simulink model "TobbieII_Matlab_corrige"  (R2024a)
settings: Solver=VariableStepAuto  StartTime=0.0  StopTime=10  RelTol=1e-3
model workspace: external: MATLAB File (data not in the file)
undefined symbols (not defined in the file or in its folder): deg, kg, m, mm, N, s, smiData, X, Y, Z
libraries: sm_lib x63, fl_lib x16, nesl_utility x9, ee_lib x2, simulink x1
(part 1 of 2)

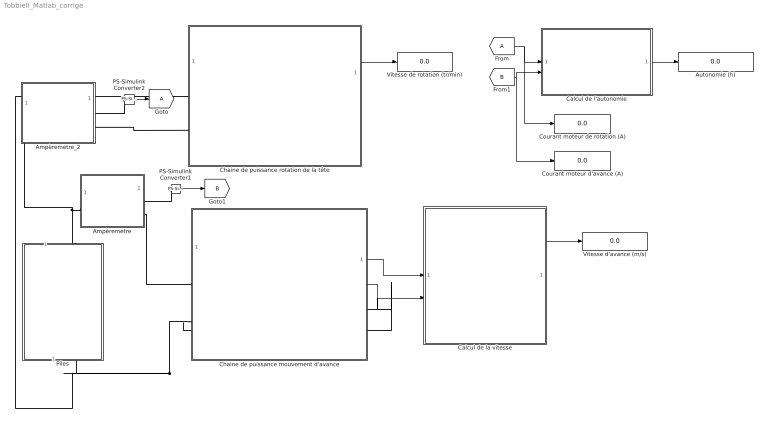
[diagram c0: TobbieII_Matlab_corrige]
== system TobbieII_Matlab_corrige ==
  Ampèremetre : Subsystem
  Ampèremetre_2 : Subsystem
  Autonomie (h) : Display
  Calcul de l'autonomie : Subsystem
  Calcul de la vitesse : Subsystem
  Chaine de puissance mouvement d'avance : Subsystem  mask{reducteur=(36*40*36*25)/(8*14*10*10)}
      mask prompts: reducteur "Rapport de réduction (1/r)"
  Chaine de puissance rotation de la tête : Subsystem  mask{reducteur=(34*32*36*32*60)/(8*14*10*14*10)}
      mask prompts: reducteur "rapport de reduction (1/r)"
  Courant moteur d'avance (A) : Display
  Courant moteur de rotation (A) : Display
  From : From
  Goto : Goto
  PS-Simulink Converter1 : nesl_utility/PS-Simulink Converter  PhysicalDomain=network_engine_domain  SubClassName=ps_output  LeftPortType=input  RightPortType=output  PseudoPeriodic=off  Frequencies=[]  VectorFormat=inherit  Unit=A  AffineConversion=off
  PS-Simulink Converter2 : nesl_utility/PS-Simulink Converter  PhysicalDomain=network_engine_domain  SubClassName=ps_output  LeftPortType=input  RightPortType=output  PseudoPeriodic=off  Frequencies=[]  VectorFormat=inherit  Unit=A  AffineConversion=off
  Piles : Subsystem  mask{tension=6}
      mask prompts: tension "Tension (V)"
  Vitesse d'avance (m/s) : Display
  Vitesse de rotation (tr/min) : Display
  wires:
  Calcul de la vitesse/1(v) -> Vitesse d'avance (m/s)/1
  PS-Simulink Converter1/1 -> [B]
  PS-Simulink Converter2/1 -> Goto/1
  Chaine de puissance mouvement d'avance/1(G2x) -> Calcul de la vitesse/1(In1)
  Chaine de puissance mouvement d'avance/2(G1x) -> Calcul de la vitesse/2(In2)
  From/1 -> Courant moteur de rotation (A)/1, Calcul de l'autonomie/1(In1)
  [B] -> Courant moteur d'avance (A)/1, Calcul de l'autonomie/2(In2)
  Calcul de l'autonomie/1(Out1) -> Autonomie (h)/1
  Chaine de puissance rotation de la tête/1(Out1) -> Vitesse de rotation (tr/min)/1
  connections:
  Ampèremetre/LConn1 -- Ampèremetre_2/LConn1 -- Piles/LConn1
  PS-Simulink Converter1/LConn1 -- Ampèremetre/RConn1
  Ampèremetre/RConn2 -- Chaine de puissance mouvement d'avance/LConn1
  PS-Simulink Converter2/LConn1 -- Ampèremetre_2/RConn1
  Ampèremetre_2/RConn2 -- Chaine de puissance rotation de la tête/LConn2
  Chaine de puissance mouvement d'avance/LConn2 -- Piles/RConn1 -- Chaine de puissance rotation de la tête/LConn1 -- Chaine de puissance mouvement d'avance/RConn1

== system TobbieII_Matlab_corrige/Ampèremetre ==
  Current Sensor : fl_lib/Electrical/Electrical Sensors/Current Sensor
  Conn1 : PMIOPort  Side=Right
  Conn2 : PMIOPort  Port=2  Side=Left
  Conn3 : PMIOPort  Port=3  Side=Right
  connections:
  Current Sensor/LConn1 -- Conn2/RConn1
  Conn1/RConn1 -- Current Sensor/RConn1
  Current Sensor/RConn2 -- Conn3/RConn1

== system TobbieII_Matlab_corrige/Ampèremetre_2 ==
  Current Sensor1 : fl_lib/Electrical/Electrical Sensors/Current Sensor
  Conn1 : PMIOPort  Side=Left
  Conn2 : PMIOPort  Port=2  Side=Right
  Conn3 : PMIOPort  Port=3  Side=Right
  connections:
  Conn2/RConn1 -- Current Sensor1/RConn1
  Current Sensor1/LConn1 -- Conn1/RConn1
  Current Sensor1/RConn2 -- Conn3/RConn1

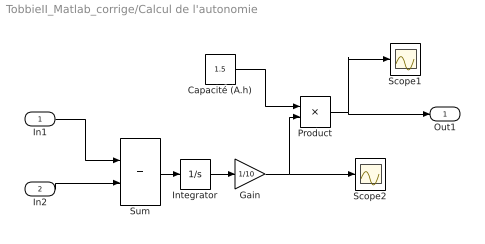
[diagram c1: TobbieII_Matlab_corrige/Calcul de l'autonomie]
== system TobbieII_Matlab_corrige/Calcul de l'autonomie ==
  In1 : Inport
  In2 : Inport  Port=2
  Capacité (A.h) : Constant  Value=1.5
  Gain : Gain  Gain=1/10
  Integrator : Integrator
  Product : Product  Inputs=*/
  Scope1 : Scope
  Scope2 : Scope
  Sum : Sum
  Out1 : Outport
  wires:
  Integrator/1 -> Gain/1
  Gain/1 -> Scope2/1, Product/2
  Capacité (A.h)/1 -> Product/1
  Sum/1 -> Integrator/1
  Product/1 -> Out1/1, Scope1/1
  In1/1 -> Sum/1
  In2/1 -> Sum/2

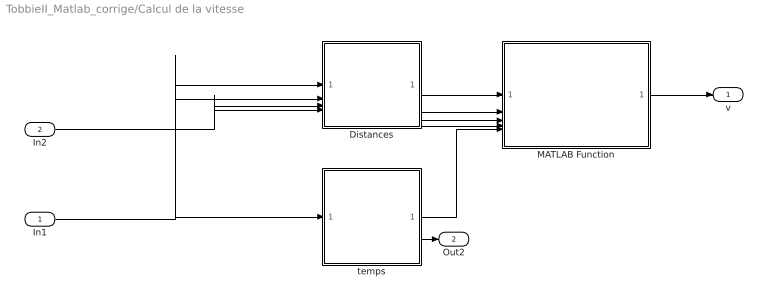
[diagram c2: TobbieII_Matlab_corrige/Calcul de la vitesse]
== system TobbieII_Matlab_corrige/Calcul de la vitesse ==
  In1 : Inport
  In2 : Inport  Port=2
  Distances : Subsystem
  MATLAB Function : MATLAB Function  TreatAsAtomicUnit=on
  temps : Subsystem
  v : Outport
  Out2 : Outport  Port=2
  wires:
  Distances/3(Out3) -> MATLAB Function/3(G2xMax)
  Distances/1(Out1) -> MATLAB Function/1(G1xMax)
  Distances/4(Out4) -> MATLAB Function/4(G2xMin)
  In2/1 -> Distances/4(In4), Distances/3(In3)
  In1/1 -> Distances/1(In1), Distances/2(In2), temps/1(U)
  temps/2(Out2) -> Out2/1
  Distances/2(Out2) -> MATLAB Function/2(G1xMin)
  temps/1(Out1) -> MATLAB Function/5(t)
  MATLAB Function/1(v) -> v/1

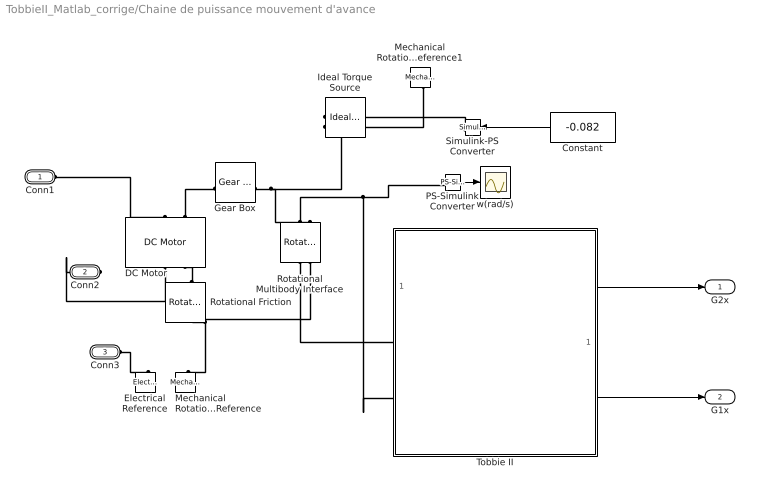
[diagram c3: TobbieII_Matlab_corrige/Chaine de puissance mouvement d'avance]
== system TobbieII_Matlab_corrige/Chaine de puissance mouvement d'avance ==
  Constant : Constant  Value=-0.082
  DC Motor : ee_lib/Electromechanical/Brushed Motors/DC Motor  field_option=ee.enum.field_option.pm  Rf=100 Ohm  Lf=1 H  Laf=0.15 H  If0=0 A  parameterization=ee.enum.dcparam_option.circuit_param  Ra=6.18 Ohm  La=2 mH  emf_or_torque=ee.enum.emf_or_torque.kv  Kv=0.0042 V*s/rad  Ki=6.876e-4 N*m/A  T_stall=0.24e-3 N*m  w_max=19100 rpm  w_rated=15000 rpm  P_rated=0.08 W  V_rated=1.5 V  lam_param=ee.enum.lam_param.damping  i_noload=0 A  V_i_noload=1.5 V  J=0.01 cm^2*g  lam=0 N*m*s/rad  speed0=0 rpm  enable_fault_armature=simscape.enum.onoff.off  rev_faulted=1 / 3  G_faulted_armature=1e-5 S  fault_trigger_armature=ee.enum.faults.faultTrigger.temporal  t_fault_armature=1 s  max_permissible_current_armature=inf A  t_fail_on_current_armature=1 s  enable_fault_field=simscape.enum.onoff.off  G_faulted_field=1e-5 S  fault_trigger_field=ee.enum.faults.faultTrigger.temporal  t_fault_field=1 s  max_permissible_current_field=inf A  t_fail_on_current_field=1 s  fault_action=simscape.enum.assert.action.none  alpha=3.93e-3 1/K  Tmeas=25 degC  thermal_mass=100 J/K  initial_temperature=25 degC
  Electrical Reference : fl_lib/Electrical/Electrical Elements/Electrical Reference
  Gear Box : fl_lib/Mechanical/Mechanisms/Gear Box  ratio=reducteur  t_in_specify=off  t_in_priority=None  t_in=0 N*m  t_in_nominal_specify=off  t_in_nominal_value=1  t_in_nominal_unit=N*m  t_out_specify=off  t_out_priority=None  t_out=0 N*m  t_out_nominal_specify=off  t_out_nominal_value=1  t_out_nominal_unit=N*m
  Ideal Torque Source : fl_lib/Mechanical/Mechanical Sources/Ideal Torque Source
  Mechanical Rotational Reference : fl_lib/Mechanical/Rotational Elements/Mechanical Rotational Reference
  Mechanical Rotational Reference1 : fl_lib/Mechanical/Rotational Elements/Mechanical Rotational Reference
  PS-Simulink Converter : nesl_utility/PS-Simulink Converter  PhysicalDomain=network_engine_domain  SubClassName=ps_output  LeftPortType=input  RightPortType=output  PseudoPeriodic=off  Frequencies=[]  VectorFormat=inherit  Unit=inherit  AffineConversion=off
  Rotational Friction : fl_lib/Mechanical/Rotational Elements/Rotational Friction  brkwy_trq=0.0029*0.007*1.8 N*m  brkwy_vel=0.01 rad/s  Col_trq=0.0029*0.005 N*m  visc_coef=0.0029*(0.14-0.007)/1365 N*m*s/rad  w_specify=off  w_priority=None  w=0 rad/s  w_nominal_specify=off  w_nominal_value=1  w_nominal_unit=rad/s  t_specify=off  t_priority=None  t=0 N*m  t_nominal_specify=off  t_nominal_value=1  t_nominal_unit=N*m
  Rotational Multibody Interface : fl_lib/Mechanical/Multibody Interfaces/Rotational Multibody Interface
  Simulink-PS Converter : nesl_utility/Simulink-PS Converter  PhysicalDomain=network_engine_domain  SubClassName=ps_input  LeftPortType=input  RightPortType=output  PseudoPeriodic=off  Frequencies=[]  NoiseDistribution=none  NoiseParameters=[]  Unit=N*m  AffineConversion=off  FilteringAndDerivatives=provide  SimscapeFilterOrder=1  InputFilterTimeConstant=0.001  UdotUserProvided=0
  Tobbie II : Subsystem
  w(rad/s) : Scope
  Conn1 : PMIOPort  Side=Left
  Conn2 : PMIOPort  Port=2  Side=Right
  Conn3 : PMIOPort  Port=3  Side=Left
  G2x : Outport
  G1x : Outport  Port=2
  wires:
  Constant/1 -> Simulink-PS Converter/1
  PS-Simulink Converter/1 -> w(rad/s)/1
  Tobbie II/2(G1x) -> G1x/1
  Tobbie II/1(G2x) -> G2x/1
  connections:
  Rotational Friction/RConn1 -- DC Motor/RConn2
  Gear Box/RConn1 -- Ideal Torque Source/LConn1 -- Rotational Multibody Interface/RConn2
  Rotational Multibody Interface/RConn1 -- PS-Simulink Converter/LConn1 -- Tobbie II/LConn2
  DC Motor/LConn2 -- Gear Box/LConn1
  Rotational Multibody Interface/LConn2 -- Rotational Friction/LConn1 -- Mechanical Rotational Reference/LConn1
  Rotational Multibody Interface/LConn1 -- Tobbie II/LConn1
  Mechanical Rotational Reference1/LConn1 -- Ideal Torque Source/RConn2
  Simulink-PS Converter/RConn1 -- Ideal Torque Source/RConn1
  Conn1/RConn1 -- DC Motor/LConn1
  DC Motor/RConn1 -- Conn2/RConn1
  Conn3/RConn1 -- Electrical Reference/LConn1

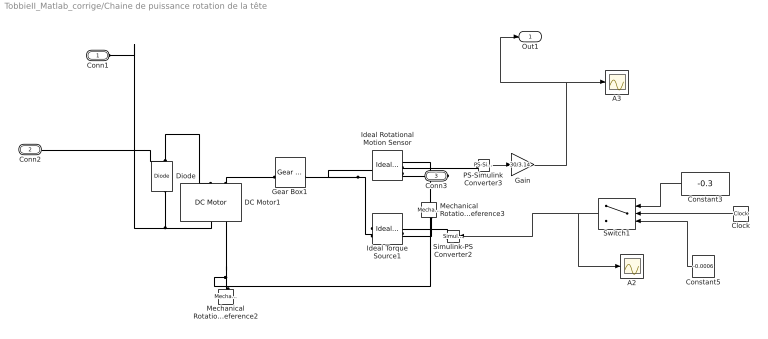
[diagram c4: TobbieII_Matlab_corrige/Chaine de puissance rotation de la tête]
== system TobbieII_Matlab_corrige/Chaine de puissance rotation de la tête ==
  A2 : Scope
  A3 : Scope
  Clock : Clock
  Constant3 : Constant  Value=-0.3
  Constant5 : Constant  Value=-0.0006
  DC Motor1 : ee_lib/Electromechanical/Brushed Motors/DC Motor  field_option=ee.enum.field_option.pm  Rf=100 Ohm  Lf=1 H  Laf=0.15 H  If0=0 A  parameterization=ee.enum.dcparam_option.circuit_param  Ra=6.18 Ohm  La=2 mH  emf_or_torque=ee.enum.emf_or_torque.kv  Kv=0.0045 V*s/rad  Ki=6.876e-4 N*m/A  T_stall=0.24e-3 N*m  w_max=19100 rpm  w_rated=15000 rpm  P_rated=0.08 W  V_rated=1.5 V  lam_param=ee.enum.lam_param.damping  i_noload=0 A  V_i_noload=1.5 V  J=0.00001 cm^2*g  lam=0 N*m*s/rad  speed0=0 rpm  enable_fault_armature=simscape.enum.onoff.off  rev_faulted=1 / 3  G_faulted_armature=1e-5 S  fault_trigger_armature=ee.enum.faults.faultTrigger.temporal  t_fault_armature=1 s  max_permissible_current_armature=inf A  t_fail_on_current_armature=1 s  enable_fault_field=simscape.enum.onoff.off  G_faulted_field=1e-5 S  fault_trigger_field=ee.enum.faults.faultTrigger.temporal  t_fault_field=1 s  max_permissible_current_field=inf A  t_fail_on_current_field=1 s  fault_action=simscape.enum.assert.action.none  alpha=3.93e-3 1/K  Tmeas=25 degC  thermal_mass=100 J/K  initial_temperature=25 degC
  Diode : fl_lib/Electrical/Electrical Elements/Diode  Vf=0.6 V  Ron=0.3 Ohm  Goff=1e-8 1/Ohm  i_specify=off  i_priority=None  i=0 A  i_nominal_specify=off  i_nominal_value=1  i_nominal_unit=A  v_specify=off  v_priority=None  v=0 V  v_nominal_specify=off  v_nominal_value=1  v_nominal_unit=V
  Gain : Gain  Gain=30/3.14
  Gear Box1 : fl_lib/Mechanical/Mechanisms/Gear Box  ratio=reducteur  t_in_specify=off  t_in_priority=None  t_in=0 N*m  t_in_nominal_specify=off  t_in_nominal_value=1  t_in_nominal_unit=N*m  t_out_specify=off  t_out_priority=None  t_out=0 N*m  t_out_nominal_specify=off  t_out_nominal_value=1  t_out_nominal_unit=N*m
  Ideal Rotational Motion Sensor : fl_lib/Mechanical/Mechanical Sensors/Ideal Rotational Motion Sensor  reference=foundation.enum.MeasurementReference.difference  acceleration_port=false  velocity_port=true  position_port=true  wrap_angle=false  offset=0 rad
  Ideal Torque Source1 : fl_lib/Mechanical/Mechanical Sources/Ideal Torque Source
  Mechanical Rotational Reference2 : fl_lib/Mechanical/Rotational Elements/Mechanical Rotational Reference
  Mechanical Rotational Reference3 : fl_lib/Mechanical/Rotational Elements/Mechanical Rotational Reference
  PS-Simulink Converter3 : nesl_utility/PS-Simulink Converter  PhysicalDomain=network_engine_domain  SubClassName=ps_output  LeftPortType=input  RightPortType=output  PseudoPeriodic=off  Frequencies=[]  VectorFormat=inherit  Unit=rad/s  AffineConversion=off
  Simulink-PS Converter2 : nesl_utility/Simulink-PS Converter  PhysicalDomain=network_engine_domain  SubClassName=ps_input  LeftPortType=input  RightPortType=output  PseudoPeriodic=off  Frequencies=[]  NoiseDistribution=none  NoiseParameters=[]  Unit=N*m  AffineConversion=off  FilteringAndDerivatives=provide  SimscapeFilterOrder=1  InputFilterTimeConstant=0.001  UdotUserProvided=0
  Switch1 : Switch  Criteria=u2 > Threshold  Threshold=7
  Conn1 : PMIOPort  Side=Left
  Conn2 : PMIOPort  Port=2  Side=Left
  Conn3 : PMIOPort  Port=3  Side=Right
  Out1 : Outport
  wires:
  Switch1/1 -> A2/1, Simulink-PS Converter2/1
  Clock/1 -> Switch1/2
  Constant5/1 -> Switch1/3
  Constant3/1 -> Switch1/1
  PS-Simulink Converter3/1 -> Gain/1
  Gain/1 -> Out1/1, A3/1
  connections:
  Diode/RConn1 -- Conn2/RConn1 -- DC Motor1/LConn1
  Ideal Torque Source1/LConn1 -- Ideal Rotational Motion Sensor/LConn1 -- Gear Box1/RConn1
  Mechanical Rotational Reference3/LConn1 -- Ideal Torque Source1/RConn2
  Mechanical Rotational Reference2/LConn1 -- DC Motor1/RConn2 -- Ideal Rotational Motion Sensor/RConn1
  Diode/LConn1 -- Conn1/RConn1 -- DC Motor1/RConn1
  PS-Simulink Converter3/LConn1 -- Ideal Rotational Motion Sensor/RConn2
  Ideal Rotational Motion Sensor/RConn3 -- Conn3/RConn1
  DC Motor1/LConn2 -- Gear Box1/LConn1
  Simulink-PS Converter2/RConn1 -- Ideal Torque Source1/RConn1

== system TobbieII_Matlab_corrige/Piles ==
  DC Voltage Source1 : fl_lib/Electrical/Electrical Sources/DC Voltage Source  v0=tension V
  Conn1 : PMIOPort  Side=Left
  Conn2 : PMIOPort  Port=2  Side=Right
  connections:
  DC Voltage Source1/RConn1 -- Conn2/RConn1
  Conn1/RConn1 -- DC Voltage Source1/LConn1

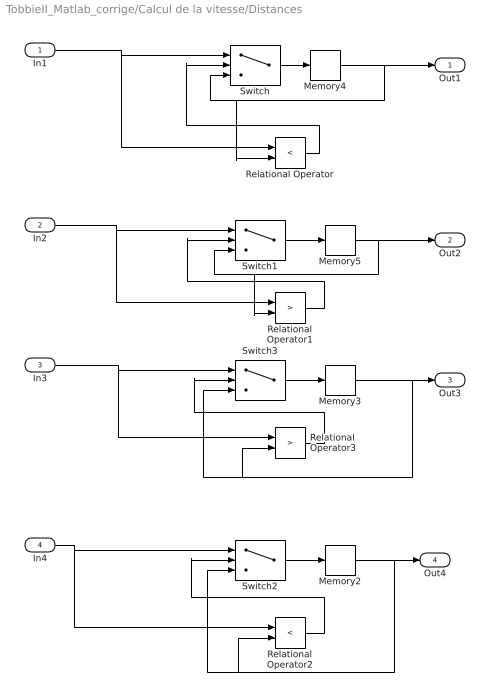
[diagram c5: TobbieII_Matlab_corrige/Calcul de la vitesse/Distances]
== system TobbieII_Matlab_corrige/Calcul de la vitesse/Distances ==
  In1 : Inport
  In2 : Inport  Port=2
  In3 : Inport  Port=3
  In4 : Inport  Port=4
  Memory2 : Memory  InitialCondition=0.09
  Memory3 : Memory  InitialCondition=0.09
  Memory4 : Memory  InitialCondition=-0.04
  Memory5 : Memory  InitialCondition=-0.04
  Relational Operator : RelationalOperator  Operator=<  OutDataTypeStr=boolean  RndMeth=Simplest
  Relational Operator1 : RelationalOperator  Operator=>  OutDataTypeStr=boolean  RndMeth=Simplest
  Relational Operator2 : RelationalOperator  Operator=<  OutDataTypeStr=boolean  RndMeth=Simplest
  Relational Operator3 : RelationalOperator  Operator=>  OutDataTypeStr=boolean  RndMeth=Simplest
  Switch{,1..3} (4 alike) : Switch  Criteria=u2 > Threshold
  Out1 : Outport
  Out2 : Outport  Port=2
  Out3 : Outport  Port=3
  Out4 : Outport  Port=4
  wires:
  Memory5/1 -> Relational Operator1/2, Switch1/3, Out2/1
  Relational Operator3/1 -> Switch3/2
  Memory3/1 -> Switch3/3, Relational Operator3/2, Out3/1
  Switch/1 -> Memory4/1
  In4/1 -> Relational Operator2/1, Switch2/1
  In1/1 -> Relational Operator/1, Switch/1
  Switch3/1 -> Memory3/1
  Memory4/1 -> Relational Operator/2, Switch/3, Out1/1
  In2/1 -> Relational Operator1/1, Switch1/1
  In3/1 -> Relational Operator3/1, Switch3/1
  Switch1/1 -> Memory5/1
  Memory2/1 -> Switch2/3, Relational Operator2/2, Out4/1
  Relational Operator/1 -> Switch/2
  Relational Operator2/1 -> Switch2/2
  Relational Operator1/1 -> Switch1/2
  Switch2/1 -> Memory2/1

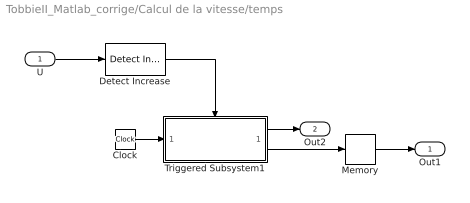
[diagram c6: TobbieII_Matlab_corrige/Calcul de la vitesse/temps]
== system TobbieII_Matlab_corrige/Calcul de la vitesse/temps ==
  U : Inport
  Clock : Clock
  Detect Increase : simulink/Logic and Bit Operations/Detect Increase  vinit=0.0  OutDataTypeStr=boolean
  Memory : Memory
  Triggered Subsystem1 : Subsystem  TreatAsAtomicUnit=on
  Out1 : Outport
  Out2 : Outport  Port=2
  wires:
  Triggered Subsystem1/2(Out2) -> Memory/1
  Memory/1 -> Out1/1
  Detect Increase/1 -> Triggered Subsystem1/Trigger
  Clock/1 -> Triggered Subsystem1/1(In1)
  Triggered Subsystem1/1(Out1) -> Out2/1
  U/1 -> Detect Increase/1

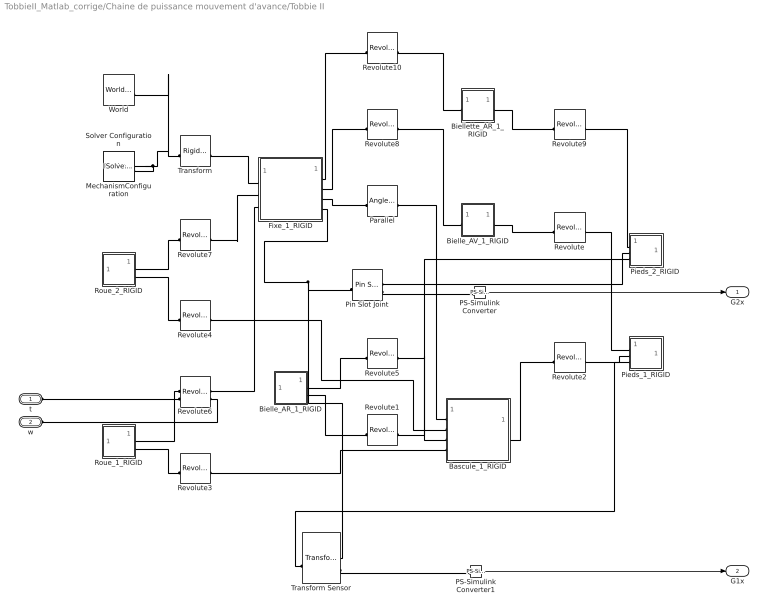
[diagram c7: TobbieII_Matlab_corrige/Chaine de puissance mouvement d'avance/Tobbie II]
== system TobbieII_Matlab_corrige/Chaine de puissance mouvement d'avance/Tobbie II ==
  Bascule_1_RIGID : Subsystem
  Bielle_AR_1_RIGID : Subsystem
  Bielle_AV_1_RIGID : Subsystem
  Biellette_AR_1_RIGID : Subsystem
  Fixe_1_RIGID : Subsystem
  MechanismConfiguration : sm_lib/Utilities/Mechanism Configuration  UniformGravity=Constant  GravityVector=[0 -9.80665 0]  GravityVectorUnits=m/s^2  LinearizationDelta=0.001  JointModeTransitionNonlinearIterations=2
  PS-Simulink Converter : nesl_utility/PS-Simulink Converter  PhysicalDomain=network_engine_domain  SubClassName=ps_output  LeftPortType=input  RightPortType=output  PseudoPeriodic=off  Frequencies=[]  VectorFormat=inherit  Unit=m  AffineConversion=off
  PS-Simulink Converter1 : nesl_utility/PS-Simulink Converter  PhysicalDomain=network_engine_domain  SubClassName=ps_output  LeftPortType=input  RightPortType=output  PseudoPeriodic=off  Frequencies=[]  VectorFormat=inherit  Unit=m  AffineConversion=off
  Parallel : sm_lib/Constraints/Angle Constraint  ConstraintType=Parallel  Angle=45  AngleUnits=deg  WrenchDir=FollowerOnBase  WrenchFrame=BaseFrame  SenseTorque=off  SenseSignedTorqueMagnitude=off
  Pieds_1_RIGID : Subsystem
  Pieds_2_RIGID : Subsystem
  Pin Slot Joint : sm_lib/Joints/Pin Slot Joint  JointMode=Normal  CompositeWrenchDir=FollowerOnBase  CompositeWrenchFrame=BaseFrame  SenseConstraintForce=off  SenseConstraintTorque=off  SenseTotalForce=off  SenseTotalTorque=off  PxPositionTargetSpecify=off  PxPositionTargetPriority=High  PxPositionTargetValue=0  PxPositionTargetValueUnits=m  PxVelocityTargetSpecify=off  PxVelocityTargetPriority=High  PxVelocityTargetValue=0  PxVelocityTargetValueUnits=m/s  PxEquilibriumPosition=0  PxEquilibriumPositionUnits=m  PxSpringStiffness=0  PxSpringStiffnessUnits=N/m  PxDampingCoefficient=0  PxDampingCoefficientUnits=N/(m/s)  PxLowerLimitSpecify=off  PxLowerLimitBound=-1  PxLowerLimitBoundUnits=m  PxLowerLimitStiffness=1e6  PxLowerLimitStiffnessUnits=N/m  PxLowerLimitDamping=1e3  PxLowerLimitDampingUnits=N/(m/s)  PxLowerLimitTransitionRegionWidth=1e-4  PxLowerLimitTransitionRegionWidthUnits=m  PxUpperLimitSpecify=off  PxUpperLimitBound=1  PxUpperLimitBoundUnits=m  PxUpperLimitStiffness=1e6  PxUpperLimitStiffnessUnits=N/m  PxUpperLimitDamping=1e3  PxUpperLimitDampingUnits=N/(m/s)  PxUpperLimitTransitionRegionWidth=1e-4  PxUpperLimitTransitionRegionWidthUnits=m  PxTorqueActuationMode=NoTorque  PxMotionActuationMode=ComputedMotion  PxSensePosition=on  PxSenseVelocity=off  PxSenseAcceleration=off  PxSenseTorqueForce=off  PxSenseLowerLimitTorqueForce=off  PxSenseUpperLimitTorqueForce=off  RzPositionTargetSpecify=off  RzPositionTargetPriority=High  RzPositionTargetValue=0  RzPositionTargetValueUnits=deg  RzVelocityTargetSpecify=off  RzVelocityTargetPriority=High  RzVelocityTargetValue=0  RzVelocityTargetValueUnits=deg/s  RzEquilibriumPosition=0  RzEquilibriumPositionUnits=deg  RzSpringStiffness=0  RzSpringStiffnessUnits=N*m/deg  RzDampingCoefficient=0  RzDampingCoefficientUnits=N*m/(deg/s)  RzLowerLimitSpecify=off  RzLowerLimitBound=-90  RzLowerLimitBoundUnits=deg  RzLowerLimitStiffness=1e4  RzLowerLimitStiffnessUnits=N*m/deg  RzLowerLimitDamping=10  RzLowerLimitDampingUnits=N*m/(deg/s)  RzLowerLimitTransitionRegionWidth=0.1  RzLowerLimitTransitionRegionWidthUnits=deg  RzUpperLimitSpecify=off  RzUpperLimitBound=90  RzUpperLimitBoundUnits=deg  RzUpperLimitStiffness=1e4  RzUpperLimitStiffnessUnits=N*m/deg  RzUpperLimitDamping=10  RzUpperLimitDampingUnits=N*m/(deg/s)  RzUpperLimitTransitionRegionWidth=0.1  RzUpperLimitTransitionRegionWidthUnits=deg  RzTorqueActuationMode=NoTorque  RzMotionActuationMode=ComputedMotion  RzSensePosition=off  RzSenseVelocity=off  RzSenseAcceleration=off  RzSenseTorqueForce=off  RzSenseLowerLimitTorqueForce=off  RzSenseUpperLimitTorqueForce=off
  Revolute : sm_lib/Joints/Revolute Joint  JointMode=Normal  CompositeWrenchDir=FollowerOnBase  CompositeWrenchFrame=BaseFrame  SenseConstraintForce=off  SenseConstraintTorque=off  SenseTotalForce=off  SenseTotalTorque=off  PositionTargetSpecify=on  PositionTargetPriority=Low  PositionTargetValue=smiData.RevoluteJoint(1).Rz.Pos  PositionTargetValueUnits=deg  VelocityTargetSpecify=off  VelocityTargetPriority=High  VelocityTargetValue=0  VelocityTargetValueUnits=deg/s  EquilibriumPosition=0  EquilibriumPositionUnits=deg  SpringStiffness=0  SpringStiffnessUnits=N*m/deg  DampingCoefficient=0  DampingCoefficientUnits=N*m/(deg/s)  LowerLimitSpecify=off  LowerLimitBound=-90  LowerLimitBoundUnits=deg  LowerLimitStiffness=1e4  LowerLimitStiffnessUnits=N*m/deg  LowerLimitDamping=10  LowerLimitDampingUnits=N*m/(deg/s)  LowerLimitTransitionRegionWidth=0.1  LowerLimitTransitionRegionWidthUnits=deg  UpperLimitSpecify=off  UpperLimitBound=90  UpperLimitBoundUnits=deg  UpperLimitStiffness=1e4  UpperLimitStiffnessUnits=N*m/deg  UpperLimitDamping=10  UpperLimitDampingUnits=N*m/(deg/s)  UpperLimitTransitionRegionWidth=0.1  UpperLimitTransitionRegionWidthUnits=deg  TorqueActuationMode=NoTorque  MotionActuationMode=ComputedMotion  SensePosition=off  SenseVelocity=off  SenseAcceleration=off  SenseTorqueForce=off  SenseLowerLimitTorqueForce=off  SenseUpperLimitTorqueForce=off
  Revolute1 : sm_lib/Joints/Revolute Joint  JointMode=Normal  CompositeWrenchDir=FollowerOnBase  CompositeWrenchFrame=BaseFrame  SenseConstraintForce=off  SenseConstraintTorque=off  SenseTotalForce=off  SenseTotalTorque=off  PositionTargetSpecify=on  PositionTargetPriority=Low  PositionTargetValue=smiData.RevoluteJoint(2).Rz.Pos  PositionTargetValueUnits=deg  VelocityTargetSpecify=off  VelocityTargetPriority=High  VelocityTargetValue=0  VelocityTargetValueUnits=deg/s  EquilibriumPosition=0  EquilibriumPositionUnits=deg  SpringStiffness=0  SpringStiffnessUnits=N*m/deg  DampingCoefficient=0  DampingCoefficientUnits=N*m/(deg/s)  LowerLimitSpecify=off  LowerLimitBound=-90  LowerLimitBoundUnits=deg  LowerLimitStiffness=1e4  LowerLimitStiffnessUnits=N*m/deg  LowerLimitDamping=10  LowerLimitDampingUnits=N*m/(deg/s)  LowerLimitTransitionRegionWidth=0.1  LowerLimitTransitionRegionWidthUnits=deg  UpperLimitSpecify=off  UpperLimitBound=90  UpperLimitBoundUnits=deg  UpperLimitStiffness=1e4  UpperLimitStiffnessUnits=N*m/deg  UpperLimitDamping=10  UpperLimitDampingUnits=N*m/(deg/s)  UpperLimitTransitionRegionWidth=0.1  UpperLimitTransitionRegionWidthUnits=deg  TorqueActuationMode=NoTorque  MotionActuationMode=ComputedMotion  SensePosition=off  SenseVelocity=off  SenseAcceleration=off  SenseTorqueForce=off  SenseLowerLimitTorqueForce=off  SenseUpperLimitTorqueForce=off
  Revolute10 : sm_lib/Joints/Revolute Joint  JointMode=Normal  CompositeWrenchDir=FollowerOnBase  CompositeWrenchFrame=BaseFrame  SenseConstraintForce=off  SenseConstraintTorque=off  SenseTotalForce=off  SenseTotalTorque=off  PositionTargetSpecify=on  PositionTargetPriority=Low  PositionTargetValue=smiData.RevoluteJoint(11).Rz.Pos  PositionTargetValueUnits=deg  VelocityTargetSpecify=off  VelocityTargetPriority=High  VelocityTargetValue=0  VelocityTargetValueUnits=deg/s  EquilibriumPosition=0  EquilibriumPositionUnits=deg  SpringStiffness=0  SpringStiffnessUnits=N*m/deg  DampingCoefficient=0  DampingCoefficientUnits=N*m/(deg/s)  LowerLimitSpecify=off  LowerLimitBound=-90  LowerLimitBoundUnits=deg  LowerLimitStiffness=1e4  LowerLimitStiffnessUnits=N*m/deg  LowerLimitDamping=10  LowerLimitDampingUnits=N*m/(deg/s)  LowerLimitTransitionRegionWidth=0.1  LowerLimitTransitionRegionWidthUnits=deg  UpperLimitSpecify=off  UpperLimitBound=90  UpperLimitBoundUnits=deg  UpperLimitStiffness=1e4  UpperLimitStiffnessUnits=N*m/deg  UpperLimitDamping=10  UpperLimitDampingUnits=N*m/(deg/s)  UpperLimitTransitionRegionWidth=0.1  UpperLimitTransitionRegionWidthUnits=deg  TorqueActuationMode=NoTorque  MotionActuationMode=ComputedMotion  SensePosition=off  SenseVelocity=off  SenseAcceleration=off  SenseTorqueForce=off  SenseLowerLimitTorqueForce=off  SenseUpperLimitTorqueForce=off
  Revolute{2,4..5,9} (4 alike) : sm_lib/Joints/Revolute Joint  JointMode=Normal  CompositeWrenchDir=FollowerOnBase  CompositeWrenchFrame=BaseFrame  SenseConstraintForce=off  SenseConstraintTorque=off  SenseTotalForce=off  SenseTotalTorque=off  PositionTargetSpecify=off  PositionTargetPriority=High  PositionTargetValue=0  PositionTargetValueUnits=deg  VelocityTargetSpecify=off  VelocityTargetPriority=High  VelocityTargetValue=0  VelocityTargetValueUnits=deg/s  EquilibriumPosition=0  EquilibriumPositionUnits=deg  SpringStiffness=0  SpringStiffnessUnits=N*m/deg  DampingCoefficient=0  DampingCoefficientUnits=N*m/(deg/s)  LowerLimitSpecify=off  LowerLimitBound=-90  LowerLimitBoundUnits=deg  LowerLimitStiffness=1e4  LowerLimitStiffnessUnits=N*m/deg  LowerLimitDamping=10  LowerLimitDampingUnits=N*m/(deg/s)  LowerLimitTransitionRegionWidth=0.1  LowerLimitTransitionRegionWidthUnits=deg  UpperLimitSpecify=off  UpperLimitBound=90  UpperLimitBoundUnits=deg  UpperLimitStiffness=1e4  UpperLimitStiffnessUnits=N*m/deg  UpperLimitDamping=10  UpperLimitDampingUnits=N*m/(deg/s)  UpperLimitTransitionRegionWidth=0.1  UpperLimitTransitionRegionWidthUnits=deg  TorqueActuationMode=NoTorque  MotionActuationMode=ComputedMotion  SensePosition=off  SenseVelocity=off  SenseAcceleration=off  SenseTorqueForce=off  SenseLowerLimitTorqueForce=off  SenseUpperLimitTorqueForce=off
  Revolute3 : sm_lib/Joints/Revolute Joint  JointMode=Normal  CompositeWrenchDir=FollowerOnBase  CompositeWrenchFrame=BaseFrame  SenseConstraintForce=off  SenseConstraintTorque=off  SenseTotalForce=off  SenseTotalTorque=off  PositionTargetSpecify=on  PositionTargetPriority=Low  PositionTargetValue=smiData.RevoluteJoint(4).Rz.Pos  PositionTargetValueUnits=deg  VelocityTargetSpecify=off  VelocityTargetPriority=High  VelocityTargetValue=0  VelocityTargetValueUnits=deg/s  EquilibriumPosition=0  EquilibriumPositionUnits=deg  SpringStiffness=0  SpringStiffnessUnits=N*m/deg  DampingCoefficient=0  DampingCoefficientUnits=N*m/(deg/s)  LowerLimitSpecify=off  LowerLimitBound=-90  LowerLimitBoundUnits=deg  LowerLimitStiffness=1e4  LowerLimitStiffnessUnits=N*m/deg  LowerLimitDamping=10  LowerLimitDampingUnits=N*m/(deg/s)  LowerLimitTransitionRegionWidth=0.1  LowerLimitTransitionRegionWidthUnits=deg  UpperLimitSpecify=off  UpperLimitBound=90  UpperLimitBoundUnits=deg  UpperLimitStiffness=1e4  UpperLimitStiffnessUnits=N*m/deg  UpperLimitDamping=10  UpperLimitDampingUnits=N*m/(deg/s)  UpperLimitTransitionRegionWidth=0.1  UpperLimitTransitionRegionWidthUnits=deg  TorqueActuationMode=NoTorque  MotionActuationMode=ComputedMotion  SensePosition=off  SenseVelocity=off  SenseAcceleration=off  SenseTorqueForce=off  SenseLowerLimitTorqueForce=off  SenseUpperLimitTorqueForce=off
  Revolute6 : sm_lib/Joints/Revolute Joint  JointMode=Normal  CompositeWrenchDir=FollowerOnBase  CompositeWrenchFrame=BaseFrame  SenseConstraintForce=off  SenseConstraintTorque=off  SenseTotalForce=off  SenseTotalTorque=off  PositionTargetSpecify=on  PositionTargetPriority=Low  PositionTargetValue=smiData.RevoluteJoint(7).Rz.Pos  PositionTargetValueUnits=deg  VelocityTargetSpecify=off  VelocityTargetPriority=High  VelocityTargetValue=0  VelocityTargetValueUnits=deg/s  EquilibriumPosition=0  EquilibriumPositionUnits=deg  SpringStiffness=0  SpringStiffnessUnits=N*m/deg  DampingCoefficient=0  DampingCoefficientUnits=N*m/(deg/s)  LowerLimitSpecify=off  LowerLimitBound=-90  LowerLimitBoundUnits=deg  LowerLimitStiffness=1e4  LowerLimitStiffnessUnits=N*m/deg  LowerLimitDamping=10  LowerLimitDampingUnits=N*m/(deg/s)  LowerLimitTransitionRegionWidth=0.1  LowerLimitTransitionRegionWidthUnits=deg  UpperLimitSpecify=off  UpperLimitBound=90  UpperLimitBoundUnits=deg  UpperLimitStiffness=1e4  UpperLimitStiffnessUnits=N*m/deg  UpperLimitDamping=10  UpperLimitDampingUnits=N*m/(deg/s)  UpperLimitTransitionRegionWidth=0.1  UpperLimitTransitionRegionWidthUnits=deg  TorqueActuationMode=InputTorque  MotionActuationMode=ComputedMotion  SensePosition=off  SenseVelocity=on  SenseAcceleration=off  SenseTorqueForce=off  SenseLowerLimitTorqueForce=off  SenseUpperLimitTorqueForce=off
  Revolute7 : sm_lib/Joints/Revolute Joint  JointMode=Normal  CompositeWrenchDir=FollowerOnBase  CompositeWrenchFrame=BaseFrame  SenseConstraintForce=off  SenseConstraintTorque=off  SenseTotalForce=off  SenseTotalTorque=off  PositionTargetSpecify=on  PositionTargetPriority=Low  PositionTargetValue=smiData.RevoluteJoint(8).Rz.Pos  PositionTargetValueUnits=deg  VelocityTargetSpecify=off  VelocityTargetPriority=High  VelocityTargetValue=0  VelocityTargetValueUnits=deg/s  EquilibriumPosition=0  EquilibriumPositionUnits=deg  SpringStiffness=0  SpringStiffnessUnits=N*m/deg  DampingCoefficient=0  DampingCoefficientUnits=N*m/(deg/s)  LowerLimitSpecify=off  LowerLimitBound=-90  LowerLimitBoundUnits=deg  LowerLimitStiffness=1e4  LowerLimitStiffnessUnits=N*m/deg  LowerLimitDamping=10  LowerLimitDampingUnits=N*m/(deg/s)  LowerLimitTransitionRegionWidth=0.1  LowerLimitTransitionRegionWidthUnits=deg  UpperLimitSpecify=off  UpperLimitBound=90  UpperLimitBoundUnits=deg  UpperLimitStiffness=1e4  UpperLimitStiffnessUnits=N*m/deg  UpperLimitDamping=10  UpperLimitDampingUnits=N*m/(deg/s)  UpperLimitTransitionRegionWidth=0.1  UpperLimitTransitionRegionWidthUnits=deg  TorqueActuationMode=NoTorque  MotionActuationMode=ComputedMotion  SensePosition=off  SenseVelocity=off  SenseAcceleration=off  SenseTorqueForce=off  SenseLowerLimitTorqueForce=off  SenseUpperLimitTorqueForce=off
  Revolute8 : sm_lib/Joints/Revolute Joint  JointMode=Normal  CompositeWrenchDir=FollowerOnBase  CompositeWrenchFrame=BaseFrame  SenseConstraintForce=off  SenseConstraintTorque=off  SenseTotalForce=off  SenseTotalTorque=off  PositionTargetSpecify=on  PositionTargetPriority=Low  PositionTargetValue=smiData.RevoluteJoint(9).Rz.Pos  PositionTargetValueUnits=deg  VelocityTargetSpecify=off  VelocityTargetPriority=High  VelocityTargetValue=0  VelocityTargetValueUnits=deg/s  EquilibriumPosition=0  EquilibriumPositionUnits=deg  SpringStiffness=0  SpringStiffnessUnits=N*m/deg  DampingCoefficient=0  DampingCoefficientUnits=N*m/(deg/s)  LowerLimitSpecify=off  LowerLimitBound=-90  LowerLimitBoundUnits=deg  LowerLimitStiffness=1e4  LowerLimitStiffnessUnits=N*m/deg  LowerLimitDamping=10  LowerLimitDampingUnits=N*m/(deg/s)  LowerLimitTransitionRegionWidth=0.1  LowerLimitTransitionRegionWidthUnits=deg  UpperLimitSpecify=off  UpperLimitBound=90  UpperLimitBoundUnits=deg  UpperLimitStiffness=1e4  UpperLimitStiffnessUnits=N*m/deg  UpperLimitDamping=10  UpperLimitDampingUnits=N*m/(deg/s)  UpperLimitTransitionRegionWidth=0.1  UpperLimitTransitionRegionWidthUnits=deg  TorqueActuationMode=NoTorque  MotionActuationMode=ComputedMotion  SensePosition=off  SenseVelocity=off  SenseAcceleration=off  SenseTorqueForce=off  SenseLowerLimitTorqueForce=off  SenseUpperLimitTorqueForce=off
  Roue_1_RIGID : Subsystem
  Roue_2_RIGID : Subsystem
  Solver Configuration : nesl_utility/Solver Configuration  PhysicalDomain=network_engine_domain  SubClassName=solver  LeftPortType=input  RightPortType=generic  Tones=[]  Harmonics=[]  SimulateNoise=off  Profile=off  UseLocalSampling=off  EnableSwitchedLinearOptims=on  FrequencyDomain=off  UseCCode=off  RelTol=0.001  AbsTol=0.001  MinStep=1e-09  ToWorkspace=off  RevertToSquareIcSolve=off  NumHomotopyIterations=100  PhasorMode=off  PhasorModeNumHarmonics=1  ConsistencySolver=NEWTON_XTOL_AFTER_FTOL  IndexReductionMethod=DerivativeReplacement  DoDC=off  ResidualTolerance=1e-09  ConsistencyTolSource=GLOBAL  ConsistencyAbsTol=0.001  ConsistencyRelTol=0.001  ConsistencyTolFactor=0.001  UseLocalSolver=off  LocalSolverChoice=NE_BACKWARD_EULER_ADVANCER  ResolveIndetEquations=on  FunctionEvalNumThread=1  LocalSolverSampleTime=0.001  DoFixedCost=off  MaxNonlinIter=3  MaxModeIter=2  ComputeImpulses=off  ImpulseIterations=2  LinearAlgebra=auto  LinearAlgebraNumThread=0  EquationFormulation=NE_TIME_EF  DelaysMemoryBudget=1024  AutomaticFiltering=on  FilteringTimeConstant=0.001  PartitionStorageMethod=AS_NEEDED  PartitionMemoryBudget=1024  PartitionMethod=ROBUST  MultibodyUseLocalSolver=off  MultibodyLocalSolverChoice=ODE1  MultibodyLocalSolverSampleTime=0.001
  Transform : sm_lib/Frames and Transforms/Rigid Transform  RotationMethod=ArbitraryAxis  FollAlignAxisA=+X  BaseAlignAxisA=+Y  FollAlignAxisB=+Y  BaseAlignAxisB=+Z  RotationStandardAxis=+Z  RotationAngle=smiData.RigidTransform(27).angle  RotationAngleUnits=rad  RotationArbitraryAxis=smiData.RigidTransform(27).axis  RotationSequenceAxes=FollowerAxes  RotationSequence=XYX  RotationSequenceAngles=[0 0 0]  RotationSequenceAnglesUnits=deg  RotationMatrix=[1 0 0;0 1 0;0 0 1]  Quaternion=[1 0 0 0]  TranslationMethod=Cartesian  TranslationCartesianOffset=smiData.RigidTransform(27).translation  TranslationCartesianOffsetUnits=mm  TranslationStandardAxis=+Z  TranslationStandardOffset=0  TranslationStandardOffsetUnits=m  TranslationROffset=0  TranslationROffsetUnits=m  TranslationThetaOffset=0  TranslationThetaOffsetUnits=deg  TranslationZOffset=0  TranslationZOffsetUnits=m
  Transform Sensor : sm_lib/Frames and Transforms/Transform Sensor  MeasurementFrame=World  RotationSequence=XYX  SenseAngle=off  SenseAxis=off  SenseQ=off  SenseR=off  SenseRotationSequence=off  SenseOmegaX=off  SenseOmegaY=off  SenseOmegaZ=off  SenseOmega=off  SenseQDot=off  SenseRDot=off  SenseRotationSequenceDot=off  SenseAlphaX=off  SenseAlphaY=off  SenseAlphaZ=off  SenseAlpha=off  SenseQDDot=off  SenseRDDot=off  SenseX=on  SenseY=off  SenseZ=off  SenseXYZ=off  SenseRad=off  SenseAzim=off  SenseDist=off  SenseInc=off  SenseXDot=off  SenseYDot=off  SenseZDot=off  SenseXYZDot=off  SenseRadDot=off  SenseAzimDot=off  SenseDistDot=off  SenseIncDot=off  SenseXDDot=off  SenseYDDot=off  SenseZDDot=off  SenseXYZDDot=off  SenseRadDDot=off  SenseAzimDDot=off  SenseDistDDot=off  SenseIncDDot=off
  World : sm_lib/Frames and Transforms/World Frame
  t : PMIOPort  Side=Left
  w : PMIOPort  Port=2  Side=Left
  G2x : Outport
  G1x : Outport  Port=2
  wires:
  PS-Simulink Converter1/1 -> G1x/1
  PS-Simulink Converter/1 -> G2x/1
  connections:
  Bascule_1_RIGID/LConn2 -- Revolute4/RConn1
  Biellette_AR_1_RIGID/RConn1 -- Revolute9/LConn1
  Revolute3/LConn1 -- Roue_1_RIGID/RConn2
  Bascule_1_RIGID/LConn4 -- Revolute3/RConn1
  Bascule_1_RIGID/LConn3 -- Revolute5/RConn1
  Bielle_AV_1_RIGID/RConn1 -- Revolute/LConn1
  Fixe_1_RIGID/RConn1 -- Revolute10/LConn1
  Bielle_AV_1_RIGID/LConn1 -- Revolute8/RConn1
  Pieds_2_RIGID/LConn3 -- Revolute1/RConn1
  Fixe_1_RIGID/LConn3 -- Revolute6/RConn1
  Transform/LConn1 -- MechanismConfiguration/RConn1 -- Solver Configuration/RConn1 -- World/RConn1
  Pieds_2_RIGID/LConn1 -- Revolute9/RConn1
  Pieds_1_RIGID/LConn2 -- Revolute2/RConn1
  Fixe_1_RIGID/RConn2 -- Revolute8/LConn1
  Fixe_1_RIGID/RConn3 -- Parallel/LConn1
  Fixe_1_RIGID/RConn4 -- Transform Sensor/RConn1 -- Pin Slot Joint/LConn1
  Bascule_1_RIGID/LConn1 -- Parallel/RConn1
  Revolute6/LConn1 -- Roue_1_RIGID/RConn1
  Bielle_AR_1_RIGID/RConn1 -- Revolute5/LConn1
  Bielle_AR_1_RIGID/RConn2 -- Revolute1/LConn1
  Fixe_1_RIGID/LConn1 -- Transform/RConn1
  Revolute7/LConn1 -- Roue_2_RIGID/RConn1
  Bascule_1_RIGID/RConn1 -- Revolute2/LConn1
  Revolute4/LConn1 -- Roue_2_RIGID/RConn2
  Pieds_1_RIGID/LConn1 -- Revolute/RConn1
  Pieds_2_RIGID/LConn2 -- Pin Slot Joint/RConn1
  Biellette_AR_1_RIGID/LConn1 -- Revolute10/RConn1
  Fixe_1_RIGID/LConn2 -- Revolute7/RConn1
  Pieds_1_RIGID/LConn3 -- Transform Sensor/LConn1
  Pin Slot Joint/RConn2 -- PS-Simulink Converter/LConn1
  Transform Sensor/RConn2 -- PS-Simulink Converter1/LConn1
  t/RConn1 -- Revolute6/LConn2
  Revolute6/RConn2 -- w/RConn1

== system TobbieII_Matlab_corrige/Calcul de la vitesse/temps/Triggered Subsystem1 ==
  In1 : Inport
  Trigger : TriggerPort  VariantControl=(inherit)
  Subtract : Sum  Inputs=+-
  Unit Delay : UnitDelay  SampleTime=-1  HasFrameUpgradeWarning=on
  Out1 : Outport
  Out2 : Outport  Port=2
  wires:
  In1/1 -> Unit Delay/1, Subtract/1, Out1/1
  Unit Delay/1 -> Subtract/2
  Subtract/1 -> Out2/1

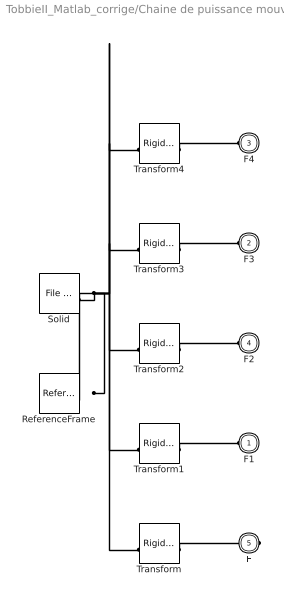
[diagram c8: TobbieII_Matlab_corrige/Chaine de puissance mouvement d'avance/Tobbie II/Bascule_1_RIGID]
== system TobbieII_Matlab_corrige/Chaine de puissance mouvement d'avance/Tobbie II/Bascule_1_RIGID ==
  ReferenceFrame : sm_lib/Frames and Transforms/Reference Frame
  Solid : sm_lib/Body Elements/File Solid  ExtGeomFileName=Bascule_Défaut_sldprt.STEP  UnitType=FromFile  ExtGeomFileUnits=m  StepReaderType=HEX  ExportConvexHullGeometry=off  InertiaType=Custom  BasedOnType=DensityFromFile  Density=1000  DensityUnits=kg/m^3  Mass=smiData.Solid(1).mass  MassUnits=kg  CenterOfMass=smiData.Solid(1).CoM  CenterOfMassUnits=mm  MomentsOfInertia=smiData.Solid(1).MoI  MomentsOfInertiaUnits=kg*mm^2  ProductsOfInertia=smiData.Solid(1).PoI  ProductsOfInertiaUnits=kg*mm^2  GraphicType=FromGeometry  MarkerShape=Sphere  MarkerSize=10  GraphicVisPropType=SimpleVisualProperties  GraphicDiffuseColor=smiData.Solid(1).color  GraphicOpacity=smiData.Solid(1).opacity  GraphicSpecularColor=[0.5 0.5 0.5 1.0]  GraphicAmbientColor=[0.15 0.15 0.15 1.0]  GraphicEmissiveColor=[0.0 0.0 0.0 1.0]  GraphicShininess=75  DoExposeReferenceFrame=on  SerializedFrames=<Frames/>
  Transform : sm_lib/Frames and Transforms/Rigid Transform  RotationMethod=ArbitraryAxis  FollAlignAxisA=+X  BaseAlignAxisA=+Y  FollAlignAxisB=+Y  BaseAlignAxisB=+Z  RotationStandardAxis=+Z  RotationAngle=smiData.RigidTransform(7).angle  RotationAngleUnits=rad  RotationArbitraryAxis=smiData.RigidTransform(7).axis  RotationSequenceAxes=FollowerAxes  RotationSequence=XYX  RotationSequenceAngles=[0 0 0]  RotationSequenceAnglesUnits=deg  RotationMatrix=[1 0 0;0 1 0;0 0 1]  Quaternion=[1 0 0 0]  TranslationMethod=Cartesian  TranslationCartesianOffset=smiData.RigidTransform(7).translation  TranslationCartesianOffsetUnits=mm  TranslationStandardAxis=+Z  TranslationStandardOffset=0  TranslationStandardOffsetUnits=m  TranslationROffset=0  TranslationROffsetUnits=m  TranslationThetaOffset=0  TranslationThetaOffsetUnits=deg  TranslationZOffset=0  TranslationZOffsetUnits=m
  Transform1 : sm_lib/Frames and Transforms/Rigid Transform  RotationMethod=ArbitraryAxis  FollAlignAxisA=+X  BaseAlignAxisA=+Y  FollAlignAxisB=+Y  BaseAlignAxisB=+Z  RotationStandardAxis=+Z  RotationAngle=smiData.RigidTransform(10).angle  RotationAngleUnits=rad  RotationArbitraryAxis=smiData.RigidTransform(10).axis  RotationSequenceAxes=FollowerAxes  RotationSequence=XYX  RotationSequenceAngles=[0 0 0]  RotationSequenceAnglesUnits=deg  RotationMatrix=[1 0 0;0 1 0;0 0 1]  Quaternion=[1 0 0 0]  TranslationMethod=Cartesian  TranslationCartesianOffset=smiData.RigidTransform(10).translation  TranslationCartesianOffsetUnits=mm  TranslationStandardAxis=+Z  TranslationStandardOffset=0  TranslationStandardOffsetUnits=m  TranslationROffset=0  TranslationROffsetUnits=m  TranslationThetaOffset=0  TranslationThetaOffsetUnits=deg  TranslationZOffset=0  TranslationZOffsetUnits=m
  Transform2 : sm_lib/Frames and Transforms/Rigid Transform  RotationMethod=ArbitraryAxis  FollAlignAxisA=+X  BaseAlignAxisA=+Y  FollAlignAxisB=+Y  BaseAlignAxisB=+Z  RotationStandardAxis=+Z  RotationAngle=smiData.RigidTransform(12).angle  RotationAngleUnits=rad  RotationArbitraryAxis=smiData.RigidTransform(12).axis  RotationSequenceAxes=FollowerAxes  RotationSequence=XYX  RotationSequenceAngles=[0 0 0]  RotationSequenceAnglesUnits=deg  RotationMatrix=[1 0 0;0 1 0;0 0 1]  Quaternion=[1 0 0 0]  TranslationMethod=Cartesian  TranslationCartesianOffset=smiData.RigidTransform(12).translation  TranslationCartesianOffsetUnits=mm  TranslationStandardAxis=+Z  TranslationStandardOffset=0  TranslationStandardOffsetUnits=m  TranslationROffset=0  TranslationROffsetUnits=m  TranslationThetaOffset=0  TranslationThetaOffsetUnits=deg  TranslationZOffset=0  TranslationZOffsetUnits=m
  Transform3 : sm_lib/Frames and Transforms/Rigid Transform  RotationMethod=ArbitraryAxis  FollAlignAxisA=+X  BaseAlignAxisA=+Y  FollAlignAxisB=+Y  BaseAlignAxisB=+Z  RotationStandardAxis=+Z  RotationAngle=smiData.RigidTransform(14).angle  RotationAngleUnits=rad  RotationArbitraryAxis=smiData.RigidTransform(14).axis  RotationSequenceAxes=FollowerAxes  RotationSequence=XYX  RotationSequenceAngles=[0 0 0]  RotationSequenceAnglesUnits=deg  RotationMatrix=[1 0 0;0 1 0;0 0 1]  Quaternion=[1 0 0 0]  TranslationMethod=Cartesian  TranslationCartesianOffset=smiData.RigidTransform(14).translation  TranslationCartesianOffsetUnits=mm  TranslationStandardAxis=+Z  TranslationStandardOffset=0  TranslationStandardOffsetUnits=m  TranslationROffset=0  TranslationROffsetUnits=m  TranslationThetaOffset=0  TranslationThetaOffsetUnits=deg  TranslationZOffset=0  TranslationZOffsetUnits=m
  Transform4 : sm_lib/Frames and Transforms/Rigid Transform  RotationMethod=ArbitraryAxis  FollAlignAxisA=+X  BaseAlignAxisA=+Y  FollAlignAxisB=+Y  BaseAlignAxisB=+Z  RotationStandardAxis=+Z  RotationAngle=smiData.RigidTransform(16).angle  RotationAngleUnits=rad  RotationArbitraryAxis=smiData.RigidTransform(16).axis  RotationSequenceAxes=FollowerAxes  RotationSequence=XYX  RotationSequenceAngles=[0 0 0]  RotationSequenceAnglesUnits=deg  RotationMatrix=[1 0 0;0 1 0;0 0 1]  Quaternion=[1 0 0 0]  TranslationMethod=Cartesian  TranslationCartesianOffset=smiData.RigidTransform(16).translation  TranslationCartesianOffsetUnits=mm  TranslationStandardAxis=+Z  TranslationStandardOffset=0  TranslationStandardOffsetUnits=m  TranslationROffset=0  TranslationROffsetUnits=m  TranslationThetaOffset=0  TranslationThetaOffsetUnits=deg  TranslationZOffset=0  TranslationZOffsetUnits=m
  F1 : PMIOPort  Side=Left
  F3 : PMIOPort  Port=2  Side=Left
  F4 : PMIOPort  Port=3  Side=Left
  F2 : PMIOPort  Port=4  Side=Left
  F : PMIOPort  Port=5  Side=Right
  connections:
  Solid/RConn1 -- ReferenceFrame/RConn1 -- Transform/LConn1 -- Transform1/LConn1 -- Transform2/LConn1 -- Transform3/LConn1 -- Transform4/LConn1
  Transform/RConn1 -- F/RConn1
  Transform1/RConn1 -- F1/RConn1
  Transform2/RConn1 -- F2/RConn1
  Transform3/RConn1 -- F3/RConn1
  Transform4/RConn1 -- F4/RConn1

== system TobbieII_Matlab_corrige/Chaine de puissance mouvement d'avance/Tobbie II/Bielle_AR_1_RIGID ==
  ReferenceFrame : sm_lib/Frames and Transforms/Reference Frame
  Solid : sm_lib/Body Elements/File Solid  ExtGeomFileName=Bielle AR_Défaut_sldprt.STEP  UnitType=FromFile  ExtGeomFileUnits=m  StepReaderType=HEX  ExportConvexHullGeometry=off  InertiaType=Custom  BasedOnType=DensityFromFile  Density=1000  DensityUnits=kg/m^3  Mass=smiData.Solid(6).mass  MassUnits=kg  CenterOfMass=smiData.Solid(6).CoM  CenterOfMassUnits=mm  MomentsOfInertia=smiData.Solid(6).MoI  MomentsOfInertiaUnits=kg*mm^2  ProductsOfInertia=smiData.Solid(6).PoI  ProductsOfInertiaUnits=kg*mm^2  GraphicType=FromGeometry  MarkerShape=Sphere  MarkerSize=10  GraphicVisPropType=SimpleVisualProperties  GraphicDiffuseColor=smiData.Solid(6).color  GraphicOpacity=smiData.Solid(6).opacity  GraphicSpecularColor=[0.5 0.5 0.5 1.0]  GraphicAmbientColor=[0.15 0.15 0.15 1.0]  GraphicEmissiveColor=[0.0 0.0 0.0 1.0]  GraphicShininess=75  DoExposeReferenceFrame=on  SerializedFrames=<Frames/>
  Transform : sm_lib/Frames and Transforms/Rigid Transform  RotationMethod=ArbitraryAxis  FollAlignAxisA=+X  BaseAlignAxisA=+Y  FollAlignAxisB=+Y  BaseAlignAxisB=+Z  RotationStandardAxis=+Z  RotationAngle=smiData.RigidTransform(5).angle  RotationAngleUnits=rad  RotationArbitraryAxis=smiData.RigidTransform(5).axis  RotationSequenceAxes=FollowerAxes  RotationSequence=XYX  RotationSequenceAngles=[0 0 0]  RotationSequenceAnglesUnits=deg  RotationMatrix=[1 0 0;0 1 0;0 0 1]  Quaternion=[1 0 0 0]  TranslationMethod=Cartesian  TranslationCartesianOffset=smiData.RigidTransform(5).translation  TranslationCartesianOffsetUnits=mm  TranslationStandardAxis=+Z  TranslationStandardOffset=0  TranslationStandardOffsetUnits=m  TranslationROffset=0  TranslationROffsetUnits=m  TranslationThetaOffset=0  TranslationThetaOffsetUnits=deg  TranslationZOffset=0  TranslationZOffsetUnits=m
  Transform1 : sm_lib/Frames and Transforms/Rigid Transform  RotationMethod=ArbitraryAxis  FollAlignAxisA=+X  BaseAlignAxisA=+Y  FollAlignAxisB=+Y  BaseAlignAxisB=+Z  RotationStandardAxis=+Z  RotationAngle=smiData.RigidTransform(15).angle  RotationAngleUnits=rad  RotationArbitraryAxis=smiData.RigidTransform(15).axis  RotationSequenceAxes=FollowerAxes  RotationSequence=XYX  RotationSequenceAngles=[0 0 0]  RotationSequenceAnglesUnits=deg  RotationMatrix=[1 0 0;0 1 0;0 0 1]  Quaternion=[1 0 0 0]  TranslationMethod=Cartesian  TranslationCartesianOffset=smiData.RigidTransform(15).translation  TranslationCartesianOffsetUnits=mm  TranslationStandardAxis=+Z  TranslationStandardOffset=0  TranslationStandardOffsetUnits=m  TranslationROffset=0  TranslationROffsetUnits=m  TranslationThetaOffset=0  TranslationThetaOffsetUnits=deg  TranslationZOffset=0  TranslationZOffsetUnits=m
  F1 : PMIOPort  Side=Right
  F : PMIOPort  Port=2  Side=Right
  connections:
  Solid/RConn1 -- ReferenceFrame/RConn1 -- Transform/LConn1 -- Transform1/LConn1
  Transform/RConn1 -- F/RConn1
  Transform1/RConn1 -- F1/RConn1

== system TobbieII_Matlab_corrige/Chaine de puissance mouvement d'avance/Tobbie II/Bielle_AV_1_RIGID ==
  ReferenceFrame : sm_lib/Frames and Transforms/Reference Frame
  Solid : sm_lib/Body Elements/File Solid  ExtGeomFileName=Bielle AV_Défaut_sldprt.STEP  UnitType=FromFile  ExtGeomFileUnits=m  StepReaderType=HEX  ExportConvexHullGeometry=off  InertiaType=Custom  BasedOnType=DensityFromFile  Density=1000  DensityUnits=kg/m^3  Mass=smiData.Solid(4).mass  MassUnits=kg  CenterOfMass=smiData.Solid(4).CoM  CenterOfMassUnits=mm  MomentsOfInertia=smiData.Solid(4).MoI  MomentsOfInertiaUnits=kg*mm^2  ProductsOfInertia=smiData.Solid(4).PoI  ProductsOfInertiaUnits=kg*mm^2  GraphicType=FromGeometry  MarkerShape=Sphere  MarkerSize=10  GraphicVisPropType=SimpleVisualProperties  GraphicDiffuseColor=smiData.Solid(4).color  GraphicOpacity=smiData.Solid(4).opacity  GraphicSpecularColor=[0.5 0.5 0.5 1.0]  GraphicAmbientColor=[0.15 0.15 0.15 1.0]  GraphicEmissiveColor=[0.0 0.0 0.0 1.0]  GraphicShininess=75  DoExposeReferenceFrame=on  SerializedFrames=<Frames/>
  Transform : sm_lib/Frames and Transforms/Rigid Transform  RotationMethod=ArbitraryAxis  FollAlignAxisA=+X  BaseAlignAxisA=+Y  FollAlignAxisB=+Y  BaseAlignAxisB=+Z  RotationStandardAxis=+Z  RotationAngle=smiData.RigidTransform(1).angle  RotationAngleUnits=rad  RotationArbitraryAxis=smiData.RigidTransform(1).axis  RotationSequenceAxes=FollowerAxes  RotationSequence=XYX  RotationSequenceAngles=[0 0 0]  RotationSequenceAnglesUnits=deg  RotationMatrix=[1 0 0;0 1 0;0 0 1]  Quaternion=[1 0 0 0]  TranslationMethod=Cartesian  TranslationCartesianOffset=smiData.RigidTransform(1).translation  TranslationCartesianOffsetUnits=mm  TranslationStandardAxis=+Z  TranslationStandardOffset=0  TranslationStandardOffsetUnits=m  TranslationROffset=0  TranslationROffsetUnits=m  TranslationThetaOffset=0  TranslationThetaOffsetUnits=deg  TranslationZOffset=0  TranslationZOffsetUnits=m
  Transform1 : sm_lib/Frames and Transforms/Rigid Transform  RotationMethod=ArbitraryAxis  FollAlignAxisA=+X  BaseAlignAxisA=+Y  FollAlignAxisB=+Y  BaseAlignAxisB=+Z  RotationStandardAxis=+Z  RotationAngle=smiData.RigidTransform(22).angle  RotationAngleUnits=rad  RotationArbitraryAxis=smiData.RigidTransform(22).axis  RotationSequenceAxes=FollowerAxes  RotationSequence=XYX  RotationSequenceAngles=[0 0 0]  RotationSequenceAnglesUnits=deg  RotationMatrix=[1 0 0;0 1 0;0 0 1]  Quaternion=[1 0 0 0]  TranslationMethod=Cartesian  TranslationCartesianOffset=smiData.RigidTransform(22).translation  TranslationCartesianOffsetUnits=mm  TranslationStandardAxis=+Z  TranslationStandardOffset=0  TranslationStandardOffsetUnits=m  TranslationROffset=0  TranslationROffsetUnits=m  TranslationThetaOffset=0  TranslationThetaOffsetUnits=deg  TranslationZOffset=0  TranslationZOffsetUnits=m
  F1 : PMIOPort  Side=Left
  F : PMIOPort  Port=2  Side=Right
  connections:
  Solid/RConn1 -- ReferenceFrame/RConn1 -- Transform/LConn1 -- Transform1/LConn1
  Transform/RConn1 -- F/RConn1
  Transform1/RConn1 -- F1/RConn1
